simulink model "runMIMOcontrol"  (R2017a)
settings: Solver=VariableStepAuto  StartTime=0.0  StopTime=150  RelTol=1e-3
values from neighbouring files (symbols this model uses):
  altu1_threshold = 0    [init.m]    (also in MISOcontrol.m = 0.2)
  altu2_threshold = 0    [init.m]    (also in MISOcontrol.m = 0.2)
  baud = 250000    [init.m]    (also in steadyState.m; MISOcontrol.m; MISO_demo.m; runSteptest.m)
  bo_c21 = 0.1    [MIMOcontrol.m]    (also in MISOcontrol.m; MISO_demo.m = 0.15)
  com = 'COM4'    [init.m]    (also in steadyState.m; MISOcontrol.m; MISO_demo.m; runSteptest.m)
  fixed_u1 = 0    [init.m]    (also in MISOcontrol.m; MISO_demo.m; SISOcontrol.m)
  fixed_u2 = 0    [init.m]    (also in MISOcontrol.m; MISO_demo.m; SISOcontrol.m)
  fixed_u3 = 0    [init.m]    (also in MISOcontrol.m; MISO_demo.m; SISOcontrol.m)
  fTf = 0.1    [init.m]    (also in steadyState.m; MISOcontrol.m; MISO_demo.m; runSteptest.m)
  fTl = 0.05    [init.m]    (also in steadyState.m; MISOcontrol.m; MISO_demo.m; runSteptest.m)
  fTt = 0.05    [init.m]    (also in steadyState.m; MISOcontrol.m; MISO_demo.m; runSteptest.m)
  step_ys1_1 = +0    (= 0)    [init.m]    (also in LightPlantMPC.m = 1; MIMOcontrol.m = -2)
  step_ys1_2 = -0    (= 0)    [init.m]    (also in LightPlantMPC.m = -1; MIMOcontrol.m)
  step_ys2_1 = 0    [init.m]    (also in LightPlantMPC.m = 5; MIMOcontrol.m = -20)
  step_ys2_2 = 0    [init.m]    (also in LightPlantMPC.m = -5; MIMOcontrol.m = 10)
  stepTime_ys1_1 = 0    [init.m]    (also in LightPlantMPC.m = 30; MIMOcontrol.m = 60)
  stepTime_ys1_2 = 0    [init.m]    (also in LightPlantMPC.m = 70; MIMOcontrol.m)
  stepTime_ys2_1 = 0    [init.m]    (also in LightPlantMPC.m = 20; MIMOcontrol.m = 30)
  stepTime_ys2_2 = 0    [init.m]    (also in LightPlantMPC.m = 50; MIMOcontrol.m = 90)
  stst_BTgain = T_est.num(2)/T_est.den(2)    [MIMOcontrol.m]
  Ts = 0.1    [init.m]    (also in steadyState.m; identification.m; MISOcontrol.m; MISO_demo.m)
  y0 = 0    [init.m]    (also in MIMOcontrol.m = 27; MISOcontrol.m = 30; MISO_demo.m = sb_T; SISOcontrol.m)
  y1_s0 = 0    [init.m]    (also in MIMOcontrol.m = stst.y(1)-y0; MISOcontrol.m)
  y2_s0 = 0    [init.m]    (also in MIMOcontrol.m = stst.y(2); MISOcontrol.m)
undefined symbols (not defined in the file or in its folder): alt_tauI11, alt_tauI21, altKc11, altKc21, Kb, Kc11, Kc12, Kc21, Kc32, maxLEDLI, tauI11, tauI12, tauI21, tauI32
libraries: simulink x12, tom_lib x1

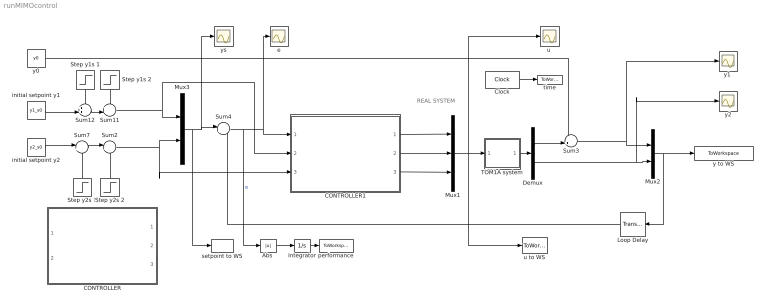
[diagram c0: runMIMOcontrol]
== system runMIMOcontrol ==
  note: REAL SYSTEM
  "Abs " : Abs  ZeroCross=off
  CONTROLLER : Subsystem  Commented=on
  CONTROLLER1 : Subsystem
  Clock : Clock
  Demux : Demux  Outputs=2
  Integrator : Integrator  ZeroCross=off
  Loop Delay : TransportDelay  DelayTime=0.1
  Mux1 : Mux  Inputs=3
  Mux2 : Mux  Inputs=2
  Mux3 : Mux  Inputs=2
  Step y1s 1 : Step  Time=stepTime_ys1_1  After=step_ys1_1  SampleTime=Ts  ZeroCross=off
  Step y1s 2 : Step  Time=stepTime_ys1_2  After=step_ys1_2  SampleTime=Ts  ZeroCross=off
  Step y2s 1 : Step  Time=stepTime_ys2_1  After=step_ys2_1  SampleTime=Ts  ZeroCross=off
  Step y2s 2 : Step  Time=stepTime_ys2_2  After=step_ys2_2  SampleTime=Ts  ZeroCross=off
  Sum11 : Sum  Inputs=++|
  Sum12 : Sum  Inputs=++|
  Sum2 : Sum  Inputs=|++
  Sum3 : Sum  Inputs=-+|
  Sum4 : Sum  Inputs=|+-
  Sum7 : Sum  Inputs=|++
  TOM1A system : Subsystem
  e : Scope
  initial setpoint y1 : Constant  Value=y1_s0  SampleTime=Ts
  initial setpoint y2 : Constant  Value=y2_s0  SampleTime=Ts
  performance : ToWorkspace  VariableName=IAE  SampleTime=Ts
  setpoint to WS : ToWorkspace  VariableName=ys  SampleTime=Ts
  time : ToWorkspace  VariableName=time  SampleTime=Ts
  "u " : Scope
  u to WS : ToWorkspace  VariableName=u  SampleTime=Ts
  y to WS : ToWorkspace  VariableName=y  SampleTime=Ts
  y0 : Constant  Value=y0  SampleTime=Ts
  "y1 " : Scope
  y2 : Scope
  ys : Scope
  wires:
  Clock/1 -> time/1
  "Abs "/1 -> Integrator/1
  TOM1A system/1(y) -> Demux/1
  Integrator/1 -> performance/1
  Mux1/1 -> u to WS/1, "u "/1, TOM1A system/1(u)
  Loop Delay/1 -> Sum4/2
  Demux/1 -> Sum3/2
  y0/1 -> Sum3/1
  initial setpoint y2/1 -> Sum7/1
  Step y2s 2/1 -> Sum2/2
  Sum7/1 -> Sum2/1
  Step y2s 1/1 -> Sum7/2
  Sum4/1 -> e/1, CONTROLLER1/1(e), "Abs "/1  "e"
  Sum3/1 -> "y1 "/1, Mux2/1
  Demux/2 -> y2/1, Mux2/2
  Mux2/1 -> Loop Delay/1, y to WS/1
  Step y1s 1/1 -> Sum12/1
  Step y1s 2/1 -> Sum11/1
  Sum12/1 -> Sum11/2
  initial setpoint y1/1 -> Sum12/2
  Sum2/1 -> CONTROLLER1/3(ys_LI), Mux3/2
  Mux3/1 -> ys/1, Sum4/1, setpoint to WS/1
  Sum11/1 -> CONTROLLER1/2(ys_T), Mux3/1
  CONTROLLER1/2(Out2) -> Mux1/2
  CONTROLLER1/3(Out3) -> Mux1/3
  CONTROLLER1/1(Out1) -> Mux1/1

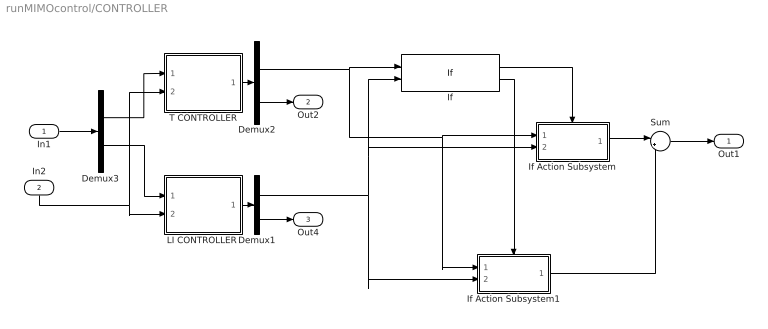
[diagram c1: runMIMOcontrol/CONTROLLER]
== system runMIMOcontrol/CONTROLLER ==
  In1 : Inport
  In2 : Inport  Port=2
  Demux1 : Demux  Outputs=2
  Demux2 : Demux  Outputs=2
  Demux3 : Demux  Outputs=2
  If : If  NumInputs=2  IfExpression=u1 > u2
  If Action Subsystem : Subsystem  TreatAsAtomicUnit=on
  If Action Subsystem1 : Subsystem  TreatAsAtomicUnit=on
  "LI CONTROLLER " : Subsystem
  Sum : Sum  Inputs=|++
  T CONTROLLER : Subsystem
  Out1 : Outport
  Out2 : Outport  Port=2
  Out4 : Outport  Port=3
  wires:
  Demux2/1 -> If Action Subsystem1/1(In1), If Action Subsystem/1(In1), If/1
  If Action Subsystem1/1(Out1) -> Sum/2
  In1/1 -> Demux3/1
  In2/1 -> "LI CONTROLLER "/2("y2s "), T CONTROLLER/2(y2s)
  Demux2/2 -> Out2/1
  Demux1/2 -> Out4/1
  "LI CONTROLLER "/1(u) -> Demux1/1
  Demux1/1 -> If Action Subsystem1/2(In2), If/2, If Action Subsystem/2(In2)
  T CONTROLLER/1(u) -> Demux2/1
  Demux3/1 -> T CONTROLLER/1(e)
  Demux3/2 -> "LI CONTROLLER "/1(e)
  If/1 -> If Action Subsystem/Action
  If/2 -> If Action Subsystem1/Action
  If Action Subsystem/1(Out1) -> Sum/1
  Sum/1 -> Out1/1

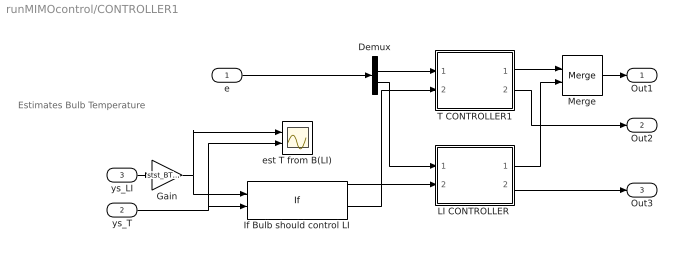
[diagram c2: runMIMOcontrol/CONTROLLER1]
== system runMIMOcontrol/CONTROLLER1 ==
  note: Estimates Bulb Temperature
  e : Inport
  ys_T : Inport  Port=2
  ys_LI : Inport  Port=3
  Demux : Demux  Outputs=2
  Gain : Gain  Gain=stst_BTgain
  If Bulb should control LI : If  NumInputs=2  IfExpression=u1 > u2  ZeroCross=off
  "LI CONTROLLER " : Subsystem
  Merge : Merge
  T CONTROLLER1 : Subsystem
  est T from B(LI) : Scope  NumInputPorts=2
  Out1 : Outport
  Out2 : Outport  Port=2
  Out3 : Outport  Port=3
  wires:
  Gain/1 -> If Bulb should control LI/1, est T from B(LI)/1
  ys_T/1 -> If Bulb should control LI/2, est T from B(LI)/2
  ys_LI/1 -> Gain/1
  If Bulb should control LI/1 -> "LI CONTROLLER "/2("sw BLI ")
  T CONTROLLER1/2(u2) -> Out2/1
  If Bulb should control LI/2 -> T CONTROLLER1/2(sw BT)
  "LI CONTROLLER "/2(u3) -> Out3/1
  e/1 -> Demux/1
  Demux/1 -> T CONTROLLER1/1(e)
  Demux/2 -> "LI CONTROLLER "/1(e)
  T CONTROLLER1/1(u1) -> Merge/1
  Merge/1 -> Out1/1
  "LI CONTROLLER "/1(u1) -> Merge/2

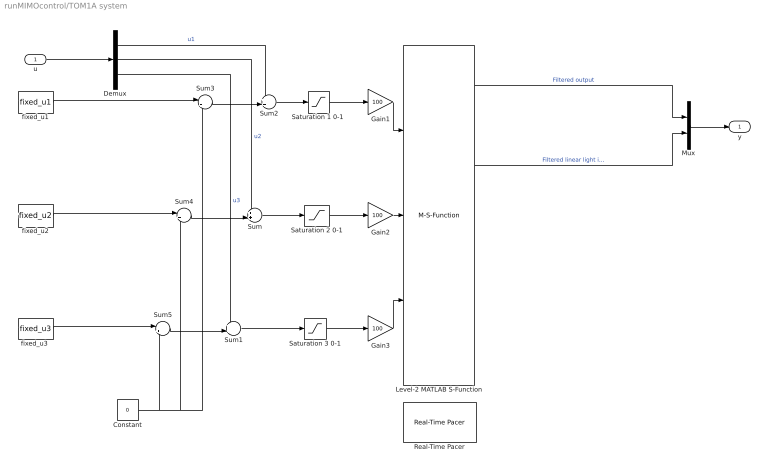
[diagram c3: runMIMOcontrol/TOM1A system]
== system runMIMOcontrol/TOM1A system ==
  u : Inport
  Constant : Constant  Value=0
  Demux : Demux  Outputs=3
  Gain1 : Gain  Gain=100
  Gain2 : Gain  Gain=100
  Gain3 : Gain  Gain=100
  Level-2 MATLAB S-Function : M-S-Function  FunctionName=tom1ar8  Parameters=Ts,com,baud,fTt,fTl,fTf
  Mux : Mux  Inputs=2
  Real-Time Pacer : tom_lib/Real-Time Pacer  simTimePerRealTime=1
  "Saturation 1 0-1 " : Saturate  UpperLimit=1  LowerLimit=0  ZeroCross=off
  Saturation 2 0-1 : Saturate  UpperLimit=1  LowerLimit=0  ZeroCross=off
  Saturation 3 0-1 : Saturate  UpperLimit=1  LowerLimit=0  ZeroCross=off
  Sum : Sum  Inputs=++|
  Sum1 : Sum  Inputs=++|
  Sum2 : Sum  Inputs=++|
  Sum3 : Sum  Inputs=|++
  Sum4 : Sum  Inputs=|++
  Sum5 : Sum  Inputs=|++
  fixed_u1 : Constant  Value=fixed_u1  SampleTime=Ts
  fixed_u2 : Constant  Value=fixed_u2  SampleTime=Ts
  "fixed_u3 " : Constant  Value=fixed_u3  SampleTime=Ts
  y : Outport
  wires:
  Level-2 MATLAB S-Function/14 -> ?  "Fan filtered  rpm"
  Level-2 MATLAB S-Function/3 -> ?  "Derivative of internal temperature"
  Level-2 MATLAB S-Function/4 -> ?  "Filtered external temperature"
  Level-2 MATLAB S-Function/13 -> ?  "Fan voltage"
  Level-2 MATLAB S-Function/11 -> ?  "Bulb voltage"
  Level-2 MATLAB S-Function/8 -> ?  "Filtered logaritmic light intensity"
  Level-2 MATLAB S-Function/1 -> ?  "Board temperature"
  Level-2 MATLAB S-Function/5 -> ?  "Derivate of external temperature"
  Level-2 MATLAB S-Function/12 -> ?  "Fan current"
  Level-2 MATLAB S-Function/9 -> ?  "Derivate of logaritmic light intensity"
  Level-2 MATLAB S-Function/16 -> ?  "Count of fan rpm"
  Level-2 MATLAB S-Function/15 -> ?  "Derivate of fan rpm"
  Level-2 MATLAB S-Function/10 -> ?  "Bulb current"
  Level-2 MATLAB S-Function/6 -> Mux/2  "Filtered linear light intensity"
  Level-2 MATLAB S-Function/7 -> ?  "Derivate of linear light intensity"
  Demux/1 -> Sum2/1  "u1"
  Demux/2 -> Sum/1  "u2"
  Demux/3 -> Sum1/1  "u3"
  u/1 -> Demux/1
  Level-2 MATLAB S-Function/2 -> Mux/1  "Filtered output"
  Mux/1 -> y/1
  fixed_u1/1 -> Sum3/1
  Sum3/1 -> Sum2/2
  Constant/1 -> Sum5/2, Sum4/2, Sum3/2
  fixed_u2/1 -> Sum4/1
  "fixed_u3 "/1 -> Sum5/1
  Sum5/1 -> Sum1/2
  Sum4/1 -> Sum/2
  Gain1/1 -> Level-2 MATLAB S-Function/1
  Gain2/1 -> Level-2 MATLAB S-Function/2
  Gain3/1 -> Level-2 MATLAB S-Function/3
  Saturation 2 0-1/1 -> Gain2/1
  Sum/1 -> Saturation 2 0-1/1
  Sum2/1 -> "Saturation 1 0-1 "/1
  Saturation 3 0-1/1 -> Gain3/1
  Sum1/1 -> Saturation 3 0-1/1
  "Saturation 1 0-1 "/1 -> Gain1/1

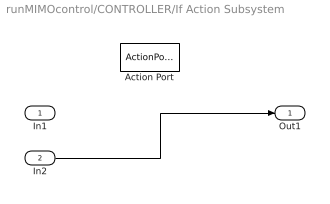
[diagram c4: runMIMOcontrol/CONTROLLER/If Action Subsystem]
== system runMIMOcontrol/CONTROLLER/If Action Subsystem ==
  In1 : Inport
  In2 : Inport  Port=2
  Action Port : ActionPort
  Out1 : Outport
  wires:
  In2/1 -> Out1/1

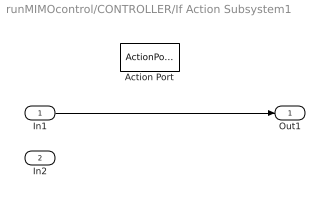
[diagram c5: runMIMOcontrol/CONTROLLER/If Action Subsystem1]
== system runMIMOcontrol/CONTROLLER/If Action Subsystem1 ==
  In1 : Inport
  In2 : Inport  Port=2
  Action Port : ActionPort
  Out1 : Outport
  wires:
  In1/1 -> Out1/1

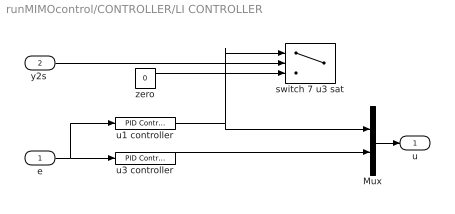
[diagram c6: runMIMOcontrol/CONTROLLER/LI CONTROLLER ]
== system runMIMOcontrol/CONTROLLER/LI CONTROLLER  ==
  e : Inport
  "y2s " : Inport  Port=2
  Mux : Mux  Inputs=2
  switch 7 u3 sat : Switch  Criteria=u2 > Threshold  Threshold=maxLEDLI
  u1 controller : simulink/Continuous/PID Controller  Controller=PI  TimeDomain=Discrete-time  SampleTime=Ts  IntegratorMethod=Forward Euler  FilterMethod=Forward Euler  Form=Parallel  UseFilter=on  ControllerParametersSource=internal  P=Kc12  I=Kc12/tauI12  D=0  N=100  InitialConditionSource=internal  InitialConditionForIntegrator=0  InitialConditionForFilter=0  ExternalReset=none  ZeroCross=off  LimitOutput=on  UpperSaturationLimit=1  LowerSaturationLimit=0  LinearizeAsGain=on  AntiWindupMode=clamping  Kb=Kb  TrackingMode=off  Kt=1  PParamMin=[]  PParamMax=[]  IParamMin=[]  IParamMax=[]  DParamMin=[]  DParamMax=[]  NParamMin=[]  NParamMax=[]  KbParamMin=[]  KbParamMax=[]  KtParamMin=[]  KtParamMax=[]  POutMin=[]  POutMax=[]  IOutMin=[]  IOutMax=[]  DOutMin=[]  DOutMax=[]  NOutMin=[]  NOutMax=[]  KbOutMin=[]  KbOutMax=[]  KtOutMin=[]  KtOutMax=[]  IntegratorOutMin=[]  IntegratorOutMax=[]  FilterOutMin=[]  FilterOutMax=[]  SumOutMin=[]  SumOutMax=[]  SumI1OutMin=[]  SumI1OutMax=[]  SumI2OutMin=[]  SumI2OutMax=[]  SumI3OutMin=[]  SumI3OutMax=[]  SumDOutMin=[]  SumDOutMax=[]  SaturationOutMin=[]  SaturationOutMax=[]  IntegratorContinuousStateAttributes=''  IntegratorStateMustResolveToSignalObject=off  IntegratorRTWStateStorageClass=Auto  FilterContinuousStateAttributes=''  FilterStateMustResolveToSignalObject=off  FilterRTWStateStorageClass=Auto  DifferentiatorICPrevScaledInput=0  DifferentiatorOutMin=[]  DifferentiatorOutMax=[]  InitialConditionSetting=State (most efficient)
  u3 controller : simulink/Continuous/PID Controller  Controller=PI  TimeDomain=Discrete-time  SampleTime=Ts  IntegratorMethod=Forward Euler  FilterMethod=Forward Euler  Form=Parallel  UseFilter=on  ControllerParametersSource=internal  P=Kc32  I=Kc32/tauI32  D=0  N=100  InitialConditionSource=internal  InitialConditionForIntegrator=0  InitialConditionForFilter=0  ExternalReset=none  ZeroCross=off  LimitOutput=on  UpperSaturationLimit=1  LowerSaturationLimit=0  LinearizeAsGain=on  AntiWindupMode=clamping  Kb=Kb  TrackingMode=off  Kt=1  PParamMin=[]  PParamMax=[]  IParamMin=[]  IParamMax=[]  DParamMin=[]  DParamMax=[]  NParamMin=[]  NParamMax=[]  KbParamMin=[]  KbParamMax=[]  KtParamMin=[]  KtParamMax=[]  POutMin=[]  POutMax=[]  IOutMin=[]  IOutMax=[]  DOutMin=[]  DOutMax=[]  NOutMin=[]  NOutMax=[]  KbOutMin=[]  KbOutMax=[]  KtOutMin=[]  KtOutMax=[]  IntegratorOutMin=[]  IntegratorOutMax=[]  FilterOutMin=[]  FilterOutMax=[]  SumOutMin=[]  SumOutMax=[]  SumI1OutMin=[]  SumI1OutMax=[]  SumI2OutMin=[]  SumI2OutMax=[]  SumI3OutMin=[]  SumI3OutMax=[]  SumDOutMin=[]  SumDOutMax=[]  SaturationOutMin=[]  SaturationOutMax=[]  IntegratorContinuousStateAttributes=''  IntegratorStateMustResolveToSignalObject=off  IntegratorRTWStateStorageClass=Auto  FilterContinuousStateAttributes=''  FilterStateMustResolveToSignalObject=off  FilterRTWStateStorageClass=Auto  DifferentiatorICPrevScaledInput=0  DifferentiatorOutMin=[]  DifferentiatorOutMax=[]  InitialConditionSetting=State (most efficient)
  zero : Constant  Value=0  SampleTime=Ts
  u : Outport
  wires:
  Mux/1 -> u/1
  u3 controller/1 -> Mux/2
  e/1 -> u1 controller/1, u3 controller/1
  u1 controller/1 -> Mux/1, switch 7 u3 sat/1
  zero/1 -> switch 7 u3 sat/3
  "y2s "/1 -> switch 7 u3 sat/2

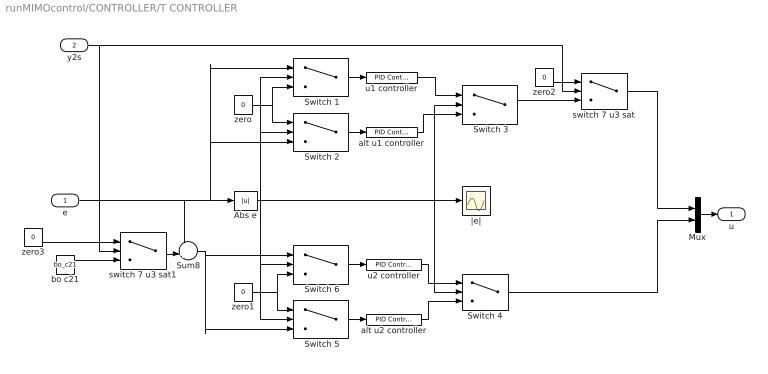
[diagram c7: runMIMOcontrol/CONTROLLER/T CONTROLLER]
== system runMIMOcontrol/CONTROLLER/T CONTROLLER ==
  e : Inport
  y2s : Inport  Port=2
  " Switch 1" : Switch  Criteria=u2 > Threshold  Threshold=altu1_threshold  ZeroCross=off
  " Switch 2" : Switch  Criteria=u2 > Threshold  Threshold=altu1_threshold  ZeroCross=off
  " Switch 3" : Switch  Criteria=u2 > Threshold  Threshold=altu1_threshold  ZeroCross=off
  " Switch 5" : Switch  Criteria=u2 > Threshold  Threshold=altu2_threshold  ZeroCross=off
  " Switch 6" : Switch  Criteria=u2 > Threshold  Threshold=altu2_threshold  ZeroCross=off
  Abs e : Abs  ZeroCross=off
  Mux : Mux  Inputs=2
  Sum8 : Sum  Inputs=++|
  Switch 4 : Switch  Criteria=u2 > Threshold  Threshold=altu2_threshold  ZeroCross=off
  alt u1 controller : simulink/Continuous/PID Controller  Controller=PI  TimeDomain=Discrete-time  SampleTime=Ts  IntegratorMethod=Forward Euler  FilterMethod=Forward Euler  Form=Parallel  UseFilter=on  ControllerParametersSource=internal  P=altKc11  I=altKc11/alt_tauI11  D=0  N=100  InitialConditionSource=internal  InitialConditionForIntegrator=0  InitialConditionForFilter=0  ExternalReset=none  ZeroCross=off  LimitOutput=on  UpperSaturationLimit=1  LowerSaturationLimit=0  LinearizeAsGain=on  AntiWindupMode=clamping  Kb=Kb  TrackingMode=off  Kt=1  PParamMin=[]  PParamMax=[]  IParamMin=[]  IParamMax=[]  DParamMin=[]  DParamMax=[]  NParamMin=[]  NParamMax=[]  KbParamMin=[]  KbParamMax=[]  KtParamMin=[]  KtParamMax=[]  POutMin=[]  POutMax=[]  IOutMin=[]  IOutMax=[]  DOutMin=[]  DOutMax=[]  NOutMin=[]  NOutMax=[]  KbOutMin=[]  KbOutMax=[]  KtOutMin=[]  KtOutMax=[]  IntegratorOutMin=[]  IntegratorOutMax=[]  FilterOutMin=[]  FilterOutMax=[]  SumOutMin=[]  SumOutMax=[]  SumI1OutMin=[]  SumI1OutMax=[]  SumI2OutMin=[]  SumI2OutMax=[]  SumI3OutMin=[]  SumI3OutMax=[]  SumDOutMin=[]  SumDOutMax=[]  SaturationOutMin=[]  SaturationOutMax=[]  IntegratorContinuousStateAttributes=''  IntegratorStateMustResolveToSignalObject=off  IntegratorRTWStateStorageClass=Auto  FilterContinuousStateAttributes=''  FilterStateMustResolveToSignalObject=off  FilterRTWStateStorageClass=Auto  DifferentiatorICPrevScaledInput=0  DifferentiatorOutMin=[]  DifferentiatorOutMax=[]  InitialConditionSetting=State (most efficient)
  alt u2 controller : simulink/Continuous/PID Controller  Controller=PI  TimeDomain=Discrete-time  SampleTime=Ts  IntegratorMethod=Forward Euler  FilterMethod=Forward Euler  Form=Parallel  UseFilter=on  ControllerParametersSource=internal  P=altKc21  I=altKc21/alt_tauI21  D=0  N=100  InitialConditionSource=internal  InitialConditionForIntegrator=0  InitialConditionForFilter=0  ExternalReset=none  ZeroCross=off  LimitOutput=on  UpperSaturationLimit=1  LowerSaturationLimit=0  LinearizeAsGain=on  AntiWindupMode=clamping  Kb=Kb  TrackingMode=off  Kt=1  PParamMin=[]  PParamMax=[]  IParamMin=[]  IParamMax=[]  DParamMin=[]  DParamMax=[]  NParamMin=[]  NParamMax=[]  KbParamMin=[]  KbParamMax=[]  KtParamMin=[]  KtParamMax=[]  POutMin=[]  POutMax=[]  IOutMin=[]  IOutMax=[]  DOutMin=[]  DOutMax=[]  NOutMin=[]  NOutMax=[]  KbOutMin=[]  KbOutMax=[]  KtOutMin=[]  KtOutMax=[]  IntegratorOutMin=[]  IntegratorOutMax=[]  FilterOutMin=[]  FilterOutMax=[]  SumOutMin=[]  SumOutMax=[]  SumI1OutMin=[]  SumI1OutMax=[]  SumI2OutMin=[]  SumI2OutMax=[]  SumI3OutMin=[]  SumI3OutMax=[]  SumDOutMin=[]  SumDOutMax=[]  SaturationOutMin=[]  SaturationOutMax=[]  IntegratorContinuousStateAttributes=''  IntegratorStateMustResolveToSignalObject=off  IntegratorRTWStateStorageClass=Auto  FilterContinuousStateAttributes=''  FilterStateMustResolveToSignalObject=off  FilterRTWStateStorageClass=Auto  DifferentiatorICPrevScaledInput=0  DifferentiatorOutMin=[]  DifferentiatorOutMax=[]  InitialConditionSetting=State (most efficient)
  bo c21 : Constant  Value=bo_c21  SampleTime=Ts
  switch 7 u3 sat : Switch  Criteria=u2 > Threshold  Threshold=maxLEDLI
  switch 7 u3 sat1 : Switch  Criteria=u2 > Threshold  Threshold=maxLEDLI
  u1 controller : simulink/Continuous/PID Controller  Controller=PI  TimeDomain=Discrete-time  SampleTime=Ts  IntegratorMethod=Forward Euler  FilterMethod=Forward Euler  Form=Parallel  UseFilter=on  ControllerParametersSource=internal  P=Kc11  I=Kc11/tauI11  D=0  N=100  InitialConditionSource=internal  InitialConditionForIntegrator=0  InitialConditionForFilter=0  ExternalReset=none  ZeroCross=off  LimitOutput=on  UpperSaturationLimit=1  LowerSaturationLimit=0  LinearizeAsGain=on  AntiWindupMode=clamping  Kb=Kb  TrackingMode=off  Kt=1  PParamMin=[]  PParamMax=[]  IParamMin=[]  IParamMax=[]  DParamMin=[]  DParamMax=[]  NParamMin=[]  NParamMax=[]  KbParamMin=[]  KbParamMax=[]  KtParamMin=[]  KtParamMax=[]  POutMin=[]  POutMax=[]  IOutMin=[]  IOutMax=[]  DOutMin=[]  DOutMax=[]  NOutMin=[]  NOutMax=[]  KbOutMin=[]  KbOutMax=[]  KtOutMin=[]  KtOutMax=[]  IntegratorOutMin=[]  IntegratorOutMax=[]  FilterOutMin=[]  FilterOutMax=[]  SumOutMin=[]  SumOutMax=[]  SumI1OutMin=[]  SumI1OutMax=[]  SumI2OutMin=[]  SumI2OutMax=[]  SumI3OutMin=[]  SumI3OutMax=[]  SumDOutMin=[]  SumDOutMax=[]  SaturationOutMin=[]  SaturationOutMax=[]  IntegratorContinuousStateAttributes=''  IntegratorStateMustResolveToSignalObject=off  IntegratorRTWStateStorageClass=Auto  FilterContinuousStateAttributes=''  FilterStateMustResolveToSignalObject=off  FilterRTWStateStorageClass=Auto  DifferentiatorICPrevScaledInput=0  DifferentiatorOutMin=[]  DifferentiatorOutMax=[]  InitialConditionSetting=State (most efficient)
  u2 controller : simulink/Continuous/PID Controller  Controller=PI  TimeDomain=Discrete-time  SampleTime=Ts  IntegratorMethod=Forward Euler  FilterMethod=Forward Euler  Form=Parallel  UseFilter=on  ControllerParametersSource=internal  P=Kc21  I=Kc21/tauI21  D=0  N=100  InitialConditionSource=internal  InitialConditionForIntegrator=0  InitialConditionForFilter=0  ExternalReset=none  ZeroCross=off  LimitOutput=on  UpperSaturationLimit=1  LowerSaturationLimit=0  LinearizeAsGain=on  AntiWindupMode=clamping  Kb=Kb  TrackingMode=off  Kt=1  PParamMin=[]  PParamMax=[]  IParamMin=[]  IParamMax=[]  DParamMin=[]  DParamMax=[]  NParamMin=[]  NParamMax=[]  KbParamMin=[]  KbParamMax=[]  KtParamMin=[]  KtParamMax=[]  POutMin=[]  POutMax=[]  IOutMin=[]  IOutMax=[]  DOutMin=[]  DOutMax=[]  NOutMin=[]  NOutMax=[]  KbOutMin=[]  KbOutMax=[]  KtOutMin=[]  KtOutMax=[]  IntegratorOutMin=[]  IntegratorOutMax=[]  FilterOutMin=[]  FilterOutMax=[]  SumOutMin=[]  SumOutMax=[]  SumI1OutMin=[]  SumI1OutMax=[]  SumI2OutMin=[]  SumI2OutMax=[]  SumI3OutMin=[]  SumI3OutMax=[]  SumDOutMin=[]  SumDOutMax=[]  SaturationOutMin=[]  SaturationOutMax=[]  IntegratorContinuousStateAttributes=''  IntegratorStateMustResolveToSignalObject=off  IntegratorRTWStateStorageClass=Auto  FilterContinuousStateAttributes=''  FilterStateMustResolveToSignalObject=off  FilterRTWStateStorageClass=Auto  DifferentiatorICPrevScaledInput=0  DifferentiatorOutMin=[]  DifferentiatorOutMax=[]  InitialConditionSetting=State (most efficient)
  zero{,1..3} (4 alike) : Constant  Value=0  SampleTime=Ts
  |e| : Scope
  u : Outport
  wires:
  e/1 -> " Switch 2"/3, " Switch 1"/1, Abs e/1, Sum8/1
  Mux/1 -> u/1
  Abs e/1 -> Switch 4/2, " Switch 3"/2, |e|/1, " Switch 1"/2, " Switch 2"/2, " Switch 5"/2, " Switch 6"/2
  bo c21/1 -> switch 7 u3 sat1/3
  alt u2 controller/1 -> Switch 4/3
  u2 controller/1 -> Switch 4/1
  Switch 4/1 -> Mux/2
  " Switch 2"/1 -> alt u1 controller/1
  " Switch 1"/1 -> u1 controller/1
  zero/1 -> " Switch 2"/1, " Switch 1"/3
  alt u1 controller/1 -> " Switch 3"/3
  u1 controller/1 -> " Switch 3"/1
  " Switch 5"/1 -> alt u2 controller/1
  " Switch 6"/1 -> u2 controller/1
  zero1/1 -> " Switch 5"/1, " Switch 6"/3
  Sum8/1 -> " Switch 5"/3, " Switch 6"/1
  y2s/1 -> switch 7 u3 sat1/2, switch 7 u3 sat/2
  switch 7 u3 sat/1 -> Mux/1
  " Switch 3"/1 -> switch 7 u3 sat/3
  zero2/1 -> switch 7 u3 sat/1
  switch 7 u3 sat1/1 -> Sum8/2
  zero3/1 -> switch 7 u3 sat1/1

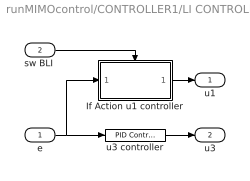
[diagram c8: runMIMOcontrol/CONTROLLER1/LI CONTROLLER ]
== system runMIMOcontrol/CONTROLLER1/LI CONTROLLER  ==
  e : Inport
  "sw BLI " : Inport  Port=2
  If Action u1 controller : Subsystem  TreatAsAtomicUnit=on
  u3 controller : simulink/Continuous/PID Controller  Controller=PI  TimeDomain=Discrete-time  SampleTime=Ts  IntegratorMethod=Forward Euler  FilterMethod=Forward Euler  Form=Parallel  UseFilter=on  ControllerParametersSource=internal  P=Kc32  I=Kc32/tauI32  D=0  N=100  InitialConditionSource=internal  InitialConditionForIntegrator=0  InitialConditionForFilter=0  ExternalReset=none  ZeroCross=off  LimitOutput=on  UpperSaturationLimit=1  LowerSaturationLimit=0  LinearizeAsGain=on  AntiWindupMode=clamping  Kb=Kb  TrackingMode=off  Kt=1  PParamMin=[]  PParamMax=[]  IParamMin=[]  IParamMax=[]  DParamMin=[]  DParamMax=[]  NParamMin=[]  NParamMax=[]  KbParamMin=[]  KbParamMax=[]  KtParamMin=[]  KtParamMax=[]  POutMin=[]  POutMax=[]  IOutMin=[]  IOutMax=[]  DOutMin=[]  DOutMax=[]  NOutMin=[]  NOutMax=[]  KbOutMin=[]  KbOutMax=[]  KtOutMin=[]  KtOutMax=[]  IntegratorOutMin=[]  IntegratorOutMax=[]  FilterOutMin=[]  FilterOutMax=[]  SumOutMin=[]  SumOutMax=[]  SumI1OutMin=[]  SumI1OutMax=[]  SumI2OutMin=[]  SumI2OutMax=[]  SumI3OutMin=[]  SumI3OutMax=[]  SumDOutMin=[]  SumDOutMax=[]  SaturationOutMin=[]  SaturationOutMax=[]  IntegratorContinuousStateAttributes=''  IntegratorStateMustResolveToSignalObject=off  IntegratorRTWStateStorageClass=Auto  FilterContinuousStateAttributes=''  FilterStateMustResolveToSignalObject=off  FilterRTWStateStorageClass=Auto  DifferentiatorICPrevScaledInput=0  DifferentiatorOutMin=[]  DifferentiatorOutMax=[]  InitialConditionSetting=State (most efficient)
  u1 : Outport
  u3 : Outport  Port=2
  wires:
  e/1 -> u3 controller/1, If Action u1 controller/1(In1)
  u3 controller/1 -> u3/1
  "sw BLI "/1 -> If Action u1 controller/Action
  If Action u1 controller/1(Out1) -> u1/1

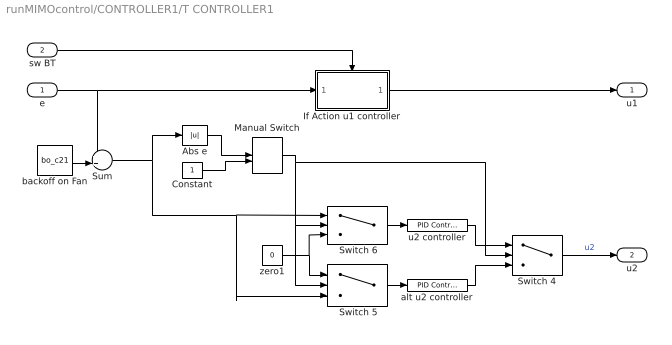
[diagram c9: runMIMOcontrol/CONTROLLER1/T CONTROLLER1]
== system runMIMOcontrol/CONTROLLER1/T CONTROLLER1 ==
  e : Inport
  sw BT : Inport  Port=2
  " Switch 5" : Switch  Criteria=u2 > Threshold  Threshold=altu2_threshold  ZeroCross=off
  " Switch 6" : Switch  Criteria=u2 > Threshold  Threshold=altu2_threshold  ZeroCross=off
  Abs e : Abs  ZeroCross=off
  Constant : Constant
  If Action u1 controller : Subsystem  TreatAsAtomicUnit=on
  Manual Switch : ManualSwitch  CurrentSetting=0
  Sum : Sum  Inputs=++|
  Switch 4 : Switch  Criteria=u2 > Threshold  Threshold=altu2_threshold  ZeroCross=off
  alt u2 controller : simulink/Continuous/PID Controller  Controller=PI  TimeDomain=Discrete-time  SampleTime=Ts  IntegratorMethod=Forward Euler  FilterMethod=Forward Euler  Form=Parallel  UseFilter=on  ControllerParametersSource=internal  P=altKc21  I=altKc21/alt_tauI21  D=0  N=100  InitialConditionSource=internal  InitialConditionForIntegrator=0  InitialConditionForFilter=0  ExternalReset=none  ZeroCross=off  LimitOutput=on  UpperSaturationLimit=1  LowerSaturationLimit=0  LinearizeAsGain=on  AntiWindupMode=clamping  Kb=Kb  TrackingMode=off  Kt=1  PParamMin=[]  PParamMax=[]  IParamMin=[]  IParamMax=[]  DParamMin=[]  DParamMax=[]  NParamMin=[]  NParamMax=[]  KbParamMin=[]  KbParamMax=[]  KtParamMin=[]  KtParamMax=[]  POutMin=[]  POutMax=[]  IOutMin=[]  IOutMax=[]  DOutMin=[]  DOutMax=[]  NOutMin=[]  NOutMax=[]  KbOutMin=[]  KbOutMax=[]  KtOutMin=[]  KtOutMax=[]  IntegratorOutMin=[]  IntegratorOutMax=[]  FilterOutMin=[]  FilterOutMax=[]  SumOutMin=[]  SumOutMax=[]  SumI1OutMin=[]  SumI1OutMax=[]  SumI2OutMin=[]  SumI2OutMax=[]  SumI3OutMin=[]  SumI3OutMax=[]  SumDOutMin=[]  SumDOutMax=[]  SaturationOutMin=[]  SaturationOutMax=[]  IntegratorContinuousStateAttributes=''  IntegratorStateMustResolveToSignalObject=off  IntegratorRTWStateStorageClass=Auto  FilterContinuousStateAttributes=''  FilterStateMustResolveToSignalObject=off  FilterRTWStateStorageClass=Auto  DifferentiatorICPrevScaledInput=0  DifferentiatorOutMin=[]  DifferentiatorOutMax=[]  InitialConditionSetting=State (most efficient)
  backoff on Fan : Constant  Value=bo_c21
  u2 controller : simulink/Continuous/PID Controller  Controller=PI  TimeDomain=Discrete-time  SampleTime=Ts  IntegratorMethod=Forward Euler  FilterMethod=Forward Euler  Form=Parallel  UseFilter=on  ControllerParametersSource=internal  P=Kc21  I=Kc21/tauI21  D=0  N=100  InitialConditionSource=internal  InitialConditionForIntegrator=0  InitialConditionForFilter=0  ExternalReset=none  ZeroCross=off  LimitOutput=on  UpperSaturationLimit=1  LowerSaturationLimit=0  LinearizeAsGain=on  AntiWindupMode=clamping  Kb=Kb  TrackingMode=off  Kt=1  PParamMin=[]  PParamMax=[]  IParamMin=[]  IParamMax=[]  DParamMin=[]  DParamMax=[]  NParamMin=[]  NParamMax=[]  KbParamMin=[]  KbParamMax=[]  KtParamMin=[]  KtParamMax=[]  POutMin=[]  POutMax=[]  IOutMin=[]  IOutMax=[]  DOutMin=[]  DOutMax=[]  NOutMin=[]  NOutMax=[]  KbOutMin=[]  KbOutMax=[]  KtOutMin=[]  KtOutMax=[]  IntegratorOutMin=[]  IntegratorOutMax=[]  FilterOutMin=[]  FilterOutMax=[]  SumOutMin=[]  SumOutMax=[]  SumI1OutMin=[]  SumI1OutMax=[]  SumI2OutMin=[]  SumI2OutMax=[]  SumI3OutMin=[]  SumI3OutMax=[]  SumDOutMin=[]  SumDOutMax=[]  SaturationOutMin=[]  SaturationOutMax=[]  IntegratorContinuousStateAttributes=''  IntegratorStateMustResolveToSignalObject=off  IntegratorRTWStateStorageClass=Auto  FilterContinuousStateAttributes=''  FilterStateMustResolveToSignalObject=off  FilterRTWStateStorageClass=Auto  DifferentiatorICPrevScaledInput=0  DifferentiatorOutMin=[]  DifferentiatorOutMax=[]  InitialConditionSetting=State (most efficient)
  zero1 : Constant  Value=0  SampleTime=Ts
  u1 : Outport
  u2 : Outport  Port=2
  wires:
  Abs e/1 -> Manual Switch/1
  alt u2 controller/1 -> Switch 4/3
  u2 controller/1 -> Switch 4/1
  Switch 4/1 -> u2/1  "u2"
  " Switch 5"/1 -> alt u2 controller/1
  " Switch 6"/1 -> u2 controller/1
  zero1/1 -> " Switch 5"/1, " Switch 6"/3
  e/1 -> Sum/1, If Action u1 controller/1(In1)
  sw BT/1 -> If Action u1 controller/Action
  If Action u1 controller/1(Out1) -> u1/1
  Sum/1 -> " Switch 5"/3, " Switch 6"/1, Abs e/1
  backoff on Fan/1 -> Sum/2
  Manual Switch/1 -> Switch 4/2, " Switch 5"/2, " Switch 6"/2
  Constant/1 -> Manual Switch/2

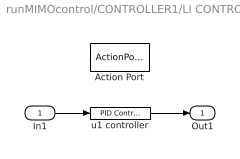
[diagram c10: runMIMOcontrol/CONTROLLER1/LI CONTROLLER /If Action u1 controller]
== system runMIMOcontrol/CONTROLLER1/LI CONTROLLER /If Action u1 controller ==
  In1 : Inport
  Action Port : ActionPort  InitializeStates=reset  ActionType=then
  u1 controller : simulink/Continuous/PID Controller  Controller=PI  TimeDomain=Discrete-time  SampleTime=-1  IntegratorMethod=Forward Euler  FilterMethod=Forward Euler  Form=Parallel  UseFilter=on  ControllerParametersSource=internal  P=Kc12  I=Kc12/tauI12  D=0  N=100  InitialConditionSource=internal  InitialConditionForIntegrator=0  InitialConditionForFilter=0  ExternalReset=none  ZeroCross=off  LimitOutput=on  UpperSaturationLimit=1  LowerSaturationLimit=0  LinearizeAsGain=on  AntiWindupMode=clamping  Kb=Kb  TrackingMode=off  Kt=1  PParamMin=[]  PParamMax=[]  IParamMin=[]  IParamMax=[]  DParamMin=[]  DParamMax=[]  NParamMin=[]  NParamMax=[]  KbParamMin=[]  KbParamMax=[]  KtParamMin=[]  KtParamMax=[]  POutMin=[]  POutMax=[]  IOutMin=[]  IOutMax=[]  DOutMin=[]  DOutMax=[]  NOutMin=[]  NOutMax=[]  KbOutMin=[]  KbOutMax=[]  KtOutMin=[]  KtOutMax=[]  IntegratorOutMin=[]  IntegratorOutMax=[]  FilterOutMin=[]  FilterOutMax=[]  SumOutMin=[]  SumOutMax=[]  SumI1OutMin=[]  SumI1OutMax=[]  SumI2OutMin=[]  SumI2OutMax=[]  SumI3OutMin=[]  SumI3OutMax=[]  SumDOutMin=[]  SumDOutMax=[]  SaturationOutMin=[]  SaturationOutMax=[]  IntegratorContinuousStateAttributes=''  IntegratorStateMustResolveToSignalObject=off  IntegratorRTWStateStorageClass=Auto  FilterContinuousStateAttributes=''  FilterStateMustResolveToSignalObject=off  FilterRTWStateStorageClass=Auto  DifferentiatorICPrevScaledInput=0  DifferentiatorOutMin=[]  DifferentiatorOutMax=[]  InitialConditionSetting=State (most efficient)
  Out1 : Outport
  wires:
  In1/1 -> u1 controller/1
  u1 controller/1 -> Out1/1

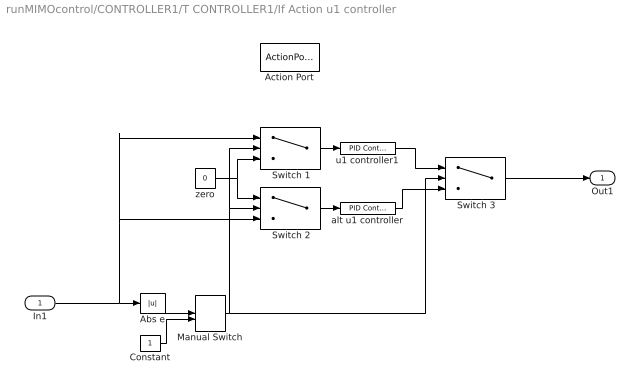
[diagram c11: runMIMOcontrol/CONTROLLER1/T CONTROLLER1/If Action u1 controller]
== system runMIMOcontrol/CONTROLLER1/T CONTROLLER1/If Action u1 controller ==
  In1 : Inport
  Action Port : ActionPort  InitializeStates=reset  ActionType=else
  " Switch 1" : Switch  Criteria=u2 > Threshold  Threshold=altu1_threshold  ZeroCross=off
  " Switch 2" : Switch  Criteria=u2 > Threshold  Threshold=altu1_threshold  ZeroCross=off
  " Switch 3" : Switch  Criteria=u2 > Threshold  Threshold=altu1_threshold  ZeroCross=off
  Abs e : Abs  ZeroCross=off
  Constant : Constant
  Manual Switch : ManualSwitch  CurrentSetting=0
  alt u1 controller : simulink/Continuous/PID Controller  Controller=PI  TimeDomain=Discrete-time  SampleTime=-1  IntegratorMethod=Forward Euler  FilterMethod=Forward Euler  Form=Parallel  UseFilter=on  ControllerParametersSource=internal  P=altKc11  I=altKc11/alt_tauI11  D=0  N=100  InitialConditionSource=internal  InitialConditionForIntegrator=0  InitialConditionForFilter=0  ExternalReset=none  ZeroCross=off  LimitOutput=on  UpperSaturationLimit=1  LowerSaturationLimit=0  LinearizeAsGain=on  AntiWindupMode=clamping  Kb=Kb  TrackingMode=off  Kt=1  PParamMin=[]  PParamMax=[]  IParamMin=[]  IParamMax=[]  DParamMin=[]  DParamMax=[]  NParamMin=[]  NParamMax=[]  KbParamMin=[]  KbParamMax=[]  KtParamMin=[]  KtParamMax=[]  POutMin=[]  POutMax=[]  IOutMin=[]  IOutMax=[]  DOutMin=[]  DOutMax=[]  NOutMin=[]  NOutMax=[]  KbOutMin=[]  KbOutMax=[]  KtOutMin=[]  KtOutMax=[]  IntegratorOutMin=[]  IntegratorOutMax=[]  FilterOutMin=[]  FilterOutMax=[]  SumOutMin=[]  SumOutMax=[]  SumI1OutMin=[]  SumI1OutMax=[]  SumI2OutMin=[]  SumI2OutMax=[]  SumI3OutMin=[]  SumI3OutMax=[]  SumDOutMin=[]  SumDOutMax=[]  SaturationOutMin=[]  SaturationOutMax=[]  IntegratorContinuousStateAttributes=''  IntegratorStateMustResolveToSignalObject=off  IntegratorRTWStateStorageClass=Auto  FilterContinuousStateAttributes=''  FilterStateMustResolveToSignalObject=off  FilterRTWStateStorageClass=Auto  DifferentiatorICPrevScaledInput=0  DifferentiatorOutMin=[]  DifferentiatorOutMax=[]  InitialConditionSetting=State (most efficient)
  u1 controller1 : simulink/Continuous/PID Controller  Controller=PI  TimeDomain=Discrete-time  SampleTime=-1  IntegratorMethod=Forward Euler  FilterMethod=Forward Euler  Form=Parallel  UseFilter=on  ControllerParametersSource=internal  P=Kc11  I=Kc11/tauI11  D=0  N=100  InitialConditionSource=internal  InitialConditionForIntegrator=0  InitialConditionForFilter=0  ExternalReset=none  ZeroCross=off  LimitOutput=on  UpperSaturationLimit=1  LowerSaturationLimit=0  LinearizeAsGain=on  AntiWindupMode=clamping  Kb=Kb  TrackingMode=off  Kt=1  PParamMin=[]  PParamMax=[]  IParamMin=[]  IParamMax=[]  DParamMin=[]  DParamMax=[]  NParamMin=[]  NParamMax=[]  KbParamMin=[]  KbParamMax=[]  KtParamMin=[]  KtParamMax=[]  POutMin=[]  POutMax=[]  IOutMin=[]  IOutMax=[]  DOutMin=[]  DOutMax=[]  NOutMin=[]  NOutMax=[]  KbOutMin=[]  KbOutMax=[]  KtOutMin=[]  KtOutMax=[]  IntegratorOutMin=[]  IntegratorOutMax=[]  FilterOutMin=[]  FilterOutMax=[]  SumOutMin=[]  SumOutMax=[]  SumI1OutMin=[]  SumI1OutMax=[]  SumI2OutMin=[]  SumI2OutMax=[]  SumI3OutMin=[]  SumI3OutMax=[]  SumDOutMin=[]  SumDOutMax=[]  SaturationOutMin=[]  SaturationOutMax=[]  IntegratorContinuousStateAttributes=''  IntegratorStateMustResolveToSignalObject=off  IntegratorRTWStateStorageClass=Auto  FilterContinuousStateAttributes=''  FilterStateMustResolveToSignalObject=off  FilterRTWStateStorageClass=Auto  DifferentiatorICPrevScaledInput=0  DifferentiatorOutMin=[]  DifferentiatorOutMax=[]  InitialConditionSetting=State (most efficient)
  zero : Constant  Value=0  SampleTime=-1
  Out1 : Outport
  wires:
  In1/1 -> Abs e/1, " Switch 2"/3, " Switch 1"/1
  u1 controller1/1 -> " Switch 3"/1
  " Switch 1"/1 -> u1 controller1/1
  " Switch 2"/1 -> alt u1 controller/1
  zero/1 -> " Switch 2"/1, " Switch 1"/3
  alt u1 controller/1 -> " Switch 3"/3
  " Switch 3"/1 -> Out1/1
  Constant/1 -> Manual Switch/2
  Abs e/1 -> Manual Switch/1
  Manual Switch/1 -> " Switch 3"/2, " Switch 2"/2, " Switch 1"/2
